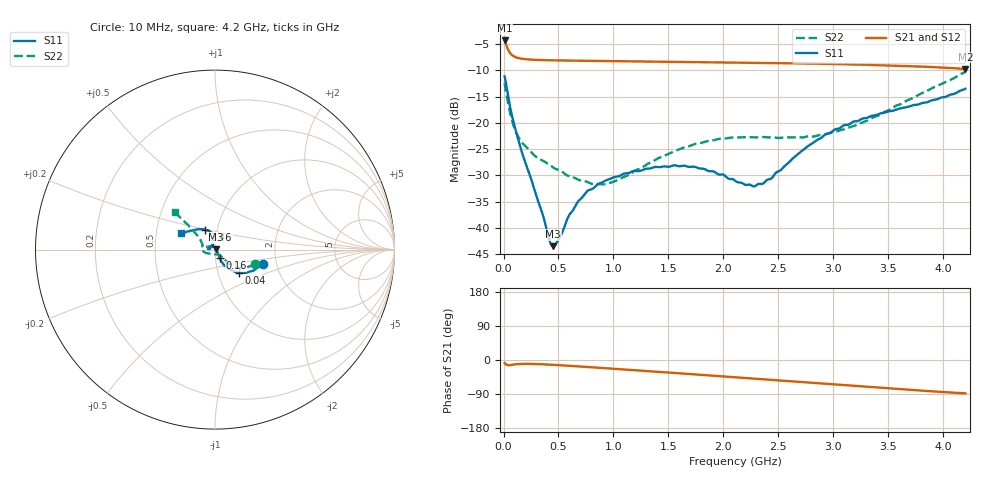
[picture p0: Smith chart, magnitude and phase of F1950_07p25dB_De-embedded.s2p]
! Integrated Device Technology
! Corporate Headquarters
! 6024 Silver Creek Valley Road
! San Jose, CA 95138  USA
! Phone:  1-408-284-8200
! Toll Free:  1-800-223-1366
! Webpage:  http://www.idt.com/
! Timing and RF Division
! 515 Groton Road, Suite 102
! Westford, MA 01886-6024
! Device:  F1950
! Description: 7-bit 0.25 dB Digital Step Attenuator
! Frequency:  150.0 -  4000.00 MHz
! Package:  4x4 mm Thin QFN Plastic Package: 24 pin
! Ports:  2 RF, 12 DC
!  Pin  1  = D0
!  Pin  2  = VDD
!  Pin  3  = Vmode
!  Pin  4  = GND
!  Pin  5  = RF1  =  Port 1
!  Pin  6  = GND
!  Pin  7  = GND
!  Pin  8  = GND
!  Pin  9  = GND
!  Pin 10  = GND
!  Pin 11  = GND
!  Pin 12  = GND
!  Pin 13  = GND
!  Pin 14  = RF2  =  Port 2
!  Pin 15  = GND
!  Pin 16  = LE
!  Pin 17  = CLK
!  Pin 18  = DATE
!  Pin 19  = D6
!  Pin 20  = D5
!  Pin 21  = D4
!  Pin 22  = D3
!  Pin 23  = D2
!  Pin 24  = D1
! State:  29
! Atten State:  7.25 dB
! Voltage:  +5.00 Volts
! Current:  Not Measured mA
! Data:  The device was measured on a the F195X evaluation board which has
!  individual transmission lines to the RF pins.  Data was collected
!  using a calibrated network analyzer.  The evaluation board was
!  de-embedded using a TRL calibration technique.
!  The reference plane is the edge of the package pin.
! Misc:  Board 2019
!  Action Tracker AT0250
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# GHz S dB R 50
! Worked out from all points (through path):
!   420 points, 10 MHz to 4.2 GHz, reference 50 ohm
!   highest |S21| = -4.31 dB at 10 MHz (marker M1); lowest = -9.7 dB at 4.2 GHz (marker M2)
!   group delay of S21, straight-line fit = 55.5 ps
!   lowest |S11| = -43.5 dB at 450 MHz (marker M3), VSWR 1.01, Z = 50.6 + j0.274 ohm
!   |S11| at or under -10 dB: start of sweep to end of sweep
!   |S22| runs from -31.7 to -10.3 dB; largest |S21 - S12| = 0.00051
!   S11 on the Smith chart (normalised r, x): 10 MHz: 1.69, -0.28; 40 MHz: 1.26, -0.33; 160 MHz: 1.05, -0.10; 3.46 GHz: 0.87, +0.20; 4.2 GHz: 0.67, +0.13
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0.01  -11.15 -16.3  -4.31 -8.1  -4.31 -8.1  -12.42 -20.1
0.04  -14.66 -43.8  -5.99 -13.7  -5.98 -13.7  -16.11 -40.2
0.1  -20.56 -60.4  -7.40 -11.7  -7.40 -11.7  -21.07 -46.0
0.16  -25.10 -60.9  -7.77 -10.4  -7.77 -10.4  -23.51 -47.0
0.35  -36.99 -35.1  -8.04 -11.3  -8.04 -11.3  -27.11 -49.9
0.42  -42.48 -2.0  -8.08 -12.2  -8.08 -12.3  -27.98 -50.6
0.45  -43.45 23.7  -8.09 -12.7  -8.09 -12.7  -28.46 -52.4
0.49  -42.55 58.6  -8.11 -13.4  -8.10 -13.4  -28.87 -55.4
0.59  -37.82 97.7  -8.14 -15.1  -8.14 -15.1  -30.09 -61.1
0.71  -34.30 114.9  -8.17 -17.4  -8.17 -17.4  -30.99 -72.6
0.77  -32.84 119.8  -8.18 -18.5  -8.18 -18.5  -31.31 -79.1
0.95  -30.78 134.0  -8.23 -22.0  -8.23 -22.0  -31.52 -105.5
1.41  -28.41 163.4  -8.34 -31.2  -8.34 -31.2  -26.68 -153.1
1.73  -28.33 175.3  -8.41 -37.8  -8.41 -37.8  -24.10 -167.5
2.11  -31.07 166.5  -8.51 -45.7  -8.51 -45.7  -22.79 -178.6
2.27  -32.07 144.2  -8.56 -49.0  -8.56 -49.0  -22.74 177.4
2.36  -31.54 129.2  -8.59 -50.9  -8.58 -50.9  -22.68 175.0
2.81  -23.87 97.3  -8.73 -60.3  -8.72 -60.3  -22.60 159.8
3.1  -20.42 103.0  -8.84 -66.5  -8.84 -66.5  -21.19 150.7
3.46  -18.08 116.7  -9.04 -74.0  -9.03 -74.0  -17.94 141.5
3.51  -17.77 118.9  -9.06 -75.0  -9.06 -75.0  -17.53 140.9
4.2  -13.49 154.1  -9.74 -88.0  -9.74 -88.0  -10.31 137.2
